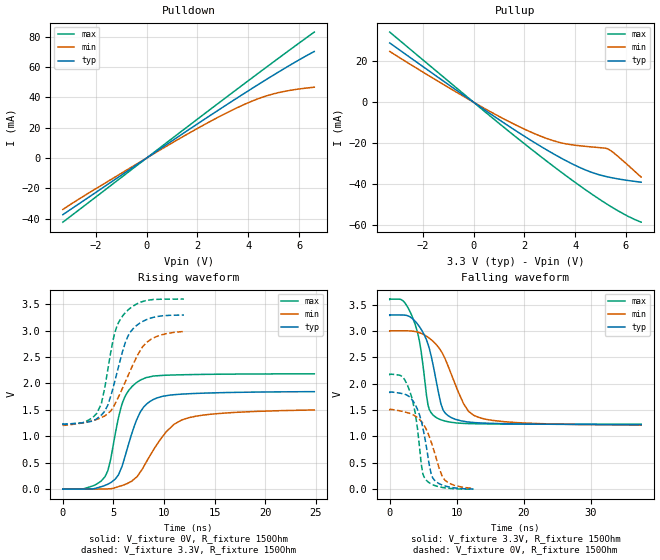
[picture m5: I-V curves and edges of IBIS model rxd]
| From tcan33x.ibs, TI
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|   rxd Model
[Model]   rxd
Model_type   Output
Polarity   Non-Inverting
Vmeas = 1.65
Vref = 1.65
Cref = 2pF
Rref = 50
|   typ   min   max
|   (nom PVT)   (fast PVT)   (slow PVT)
C_comp   4.397e-13   2.413e-13   9.068e-13
| Where nom  PVT is Nominal Process, 3.3V, 27C
|   Fast PVT is Strong Process,  3.6V, -40C
|   Slow PVT is Weak Process,   3V, 150C
[Voltage Range]   3.3   3   3.6
|Junction Temperature
[Temperature Range]   27   150   -40
[Pullup Reference]   3.3   3   3.6
[Pulldown Reference]   0   0   0
[Power Clamp Reference]   3.3   3   3.6
[GND Clamp Reference]   0   0   0
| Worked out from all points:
|   slope of the pulldown table from 0 to 0.495 V, typ, clamps not added: 87.6 ohm
|   slope of the pullup table from 0 to 0.495 V, typ, clamps not added: 115 ohm
|   falling waveform, V_fixture 3.3V, R_fixture 150Ohm: 20-80 % time 2.3ns typ, 3.74ns min, 1.79ns max; typ from 3.3 V to 1.23 V
|   rising waveform, V_fixture 0V, R_fixture 150Ohm: 20-80 % time 2ns typ, 3.27ns min, 1.57ns max; typ from 0 V to 1.84 V
|   rising waveform, V_fixture 3.3V, R_fixture 150Ohm: 20-80 % time 1.88ns typ, 2.66ns min, 1.53ns max; typ from 1.23 V to 3.29 V
|   falling waveform, V_fixture 0V, R_fixture 150Ohm: 20-80 % time 1.79ns typ, 2.5ns min, 1.48ns max; typ from 1.84 V to 0.003 V
[Pulldown]
|   Voltage   I(typ)   I(min)   I(max)
-3.3V     -37.31mA   -33.89mA   -42.28mA
-2.445V   -27.67mA   -24.71mA   -31.35mA
901.2mV   10.24mA    9.004mA    11.63mA
2.258V    25.39mA    21.92mA    28.96mA
3.45V     38.41mA    32.27mA    44.05mA
4.191V    46.33mA    37.82mA    53.36mA
4.93V     54.04mA    42.03mA    62.58mA
5.673V    61.53mA    44.7mA     71.76mA
6.6V      70.27mA    46.7mA     83.04mA
[Pullup]
|   Voltage   I(typ)   I(min)   I(max)
-3.3V     28.94mA    24.8mA     34.24mA
-1.14V    9.9mA      8.308mA    11.82mA
858mV     -7.349mA   -5.994mA   -8.881mA
2.222V    -18.39mA   -14.43mA   -22.48mA
3.295V    -26.3mA    -19.4mA    -32.76mA
3.636V    -28.59mA   -20.37mA   -35.92mA
4.343V    -32.81mA   -21.53mA   -42.26mA
4.927V    -35.43mA   -22.2mA    -47.22mA
5.286V    -36.54mA   -22.86mA   -50.09mA
5.67V     -37.47mA   -26.33mA   -52.98mA
6.095V    -38.31mA   -30.97mA   -55.87mA
6.6V      -39.11mA   -36.64mA   -58.67mA
[Ramp]
R_load = 150
|   typ   min   max
dV/dt_r   1.11021/2.01095e-09   0.912986/3.3577e-09   1.30999/1.56942e-09
dV/dt_f   1.24516/2.29933e-09   1.07594/3.7634e-09   1.42177/1.78899e-09
[Falling Waveform]
V_fixture = 3.3V
V_fixture_min = 3V
V_fixture_max = 3.6V
R_fixture = 150Ohm
|   Time   V(typ)   V(min)   V(max)
0s        3.3V       3V         3.6V
1.989ns   3.302V     3.003V     3.572V
3.34ns    3.239V     2.997V     3.279V
4.443ns   3.08V      2.966V     2.803V
5.716ns   2.746V     2.881V     1.594V
7.272ns   1.834V     2.692V     1.336V
8.589ns   1.407V     2.373V     1.283V
11.01ns   1.288V     1.625V     1.248V
13.17ns   1.259V     1.367V     1.24V
37.52ns   1.226V     1.215V     1.231V
[Rising Waveform]
V_fixture = 0V
V_fixture_min = 0V
V_fixture_max = 0V
R_fixture = 150Ohm
|   Time   V(typ)   V(min)   V(max)
0s        1.065nV    218.1nV    33.63pV
2.24ns    -99.28uV   -1.283mV   15.66mV
4.161ns   69.45mV    1.516mV    234.2mV
4.709ns   120.4mV    6.216mV    548.9mV
5.483ns   266.1mV    45.13mV    1.341V
5.908ns   466.2mV    71.14mV    1.644V
7.668ns   1.464V     328.1mV    2.064V
10.24ns   1.768V     1.09V      2.156V
11.76ns   1.798V     1.309V     2.164V
24.84ns   1.845V     1.498V     2.182V
[Rising Waveform]
V_fixture = 3.3V
V_fixture_min = 3V
V_fixture_max = 3.6V
R_fixture = 150Ohm
|   Time   V(typ)   V(min)   V(max)
0s        1.225V     1.207V     1.23V
1.989ns   1.256V     1.255V     1.258V
3.34ns    1.33V      1.319V     1.431V
3.8ns     1.401V     1.354V     1.612V
4.428ns   1.582V     1.429V     2.244V
5.11ns    2.024V     1.596V     2.944V
6.328ns   2.848V     2.099V     3.37V
6.959ns   3.04V      2.368V     3.467V
8.278ns   3.209V     2.778V     3.571V
11.96ns   3.295V     2.982V     3.597V
[Falling Waveform]
V_fixture = 0V
V_fixture_min = 0V
V_fixture_max = 0V
R_fixture = 150Ohm
|   Time   V(typ)   V(min)   V(max)
0s        1.842V     1.511V     2.179V
3.033ns   1.74V      1.435V     1.844V
3.8ns     1.604V     1.387V     1.45V
4.428ns   1.419V     1.323V     822.5mV
4.939ns   1.163V     1.249V     292.8mV
5.309ns   921.9mV    1.172V     194.4mV
6.191ns   282mV      893.1mV    99.54mV
6.719ns   165.8mV    682.5mV    70.49mV
8.278ns   59.9mV     165.9mV    25.34mV
12.48ns   3.479mV    14.7mV     1.034mV
